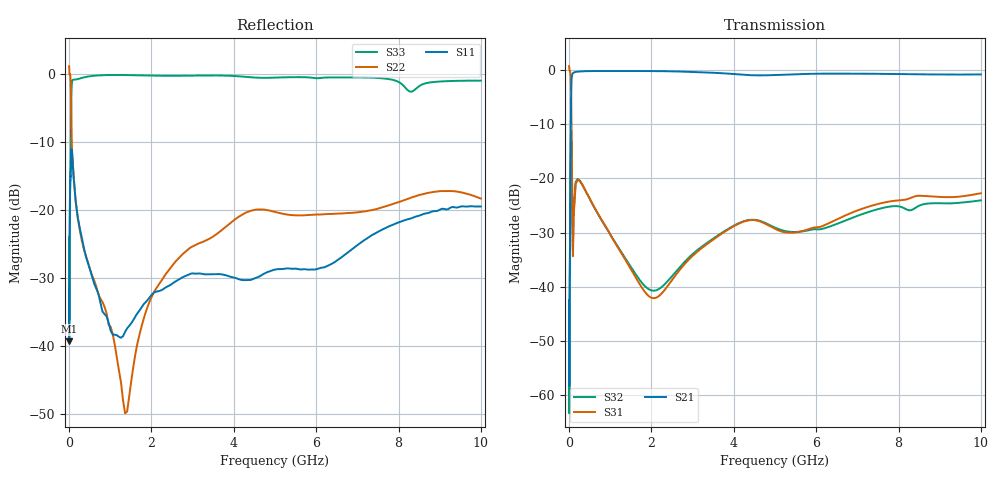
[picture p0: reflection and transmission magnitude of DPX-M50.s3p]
! MARKI MICROWAVE INC.
! Email:  info@markimicrowave.com  Phone:  408-778-4200
! Model Number:  DPX-M50  Date:  06/10
! Filename:		DPX-M50.S3P  Version: 1.0
! Description:  3-port S-parameter data for Diplexer DPX-M50
! Frequency Range: 	10 MHz to 10 GHz
! Port Configuration:	PORT 1: COMMON, PORT 2: HIGH PASS, PORT 3: LOW PASS
! Note:  S-Parameters include Test Fixture
! S3P File: Measurements: Mag<S11> Ang<S11> Mag<S12> Ang<S12> Mag<S13> Ang<S13>! row 1
!  Mag<S21> Ang<S21> Mag<S22> Ang<S22> Mag<S23> Ang<S23>! row 2
!  Mag<S31> Ang<S31> Mag<S32> Ang<S32> Mag<S33> Ang<S33>! row 3
# GHz S dB R 50
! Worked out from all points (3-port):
!   299 points, 1 MHz to 10 GHz, reference 50 ohm
!   strongest paths, dB at 1 MHz, 75 MHz, 2.56 GHz, 6.31 GHz, 10 GHz:
!     S21: -42.5, -0.9, -0.3, -0.7, -0.8
!     S31: 0.7, -22.9, -38.1, -28.3, -22.7
!     S32: -42.7, -21.6, -37.5, -28.9, -24.0
!   lowest |S11| = -39.4 dB at 5 MHz (marker M1), VSWR 1.02, Z = 50.2 - j1.06 ohm
!   |S11| at or under -10 dB: start of sweep to end of sweep
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0.001  -31.54 7.1  -41.37 55.9  0.64 -2.4
       -42.52 51.1  1.14 0.9  -39.61 21.9
       0.71 -2.4  -42.73 22.6  -24.06 74.0
0.005  -39.37 -79.2  -48.40 47.1  0.24 -9.7
       -50.64 36.7  0.48 -8.4  -45.73 10.8
       0.30 -9.5  -52.59 11.9  -29.96 59.6
0.045  -13.50 33.0  -8.20 -158.5  -2.44 -114.3
       -8.21 -158.5  -2.40 -131.9  -11.90 82.9
       -2.44 -114.2  -11.89 83.0  -8.80 -94.9
0.089  -13.25 174.9  -0.63 85.2  -33.60 -106.1
       -0.63 85.2  -12.84 -171.8  -32.40 -20.1
       -33.59 -106.0  -32.38 -20.2  -0.88 179.7
0.26  -22.72 116.1  -0.26 21.5  -20.48 -43.4
      -0.27 21.5  -22.97 126.3  -20.40 -18.7
      -20.48 -43.3  -20.40 -18.6  -0.68 88.7
1.01  -37.80 113.3  -0.17 -21.4  -30.49 -85.7
      -0.18 -21.4  -37.24 57.3  -30.47 -81.3
      -30.49 -85.7  -30.46 -81.2  -0.16 0.0
1.41  -37.46 157.4  -0.17 -34.9  -35.56 -87.4
      -0.18 -34.9  -49.69 126.5  -35.27 -84.7
      -35.56 -87.4  -35.27 -84.6  -0.17 -20.4
2.96  -29.39 177.2  -0.36 -82.8  -34.57 -11.0
      -0.36 -82.8  -25.51 131.2  -34.23 -25.1
      -34.57 -11.0  -34.23 -25.1  -0.26 -83.2
5.01  -28.79 -29.4  -0.93 -138.1  -29.34 -80.5
      -0.93 -138.1  -20.33 20.1  -29.11 -103.8
      -29.34 -80.6  -29.11 -103.8  -0.55 -156.2
10  -19.52 120.3  -0.82 81.6  -22.72 178.1
    -0.82 81.6  -18.36 -124.7  -24.04 134.2
    -22.73 178.1  -24.04 134.2  -1.00 55.1
